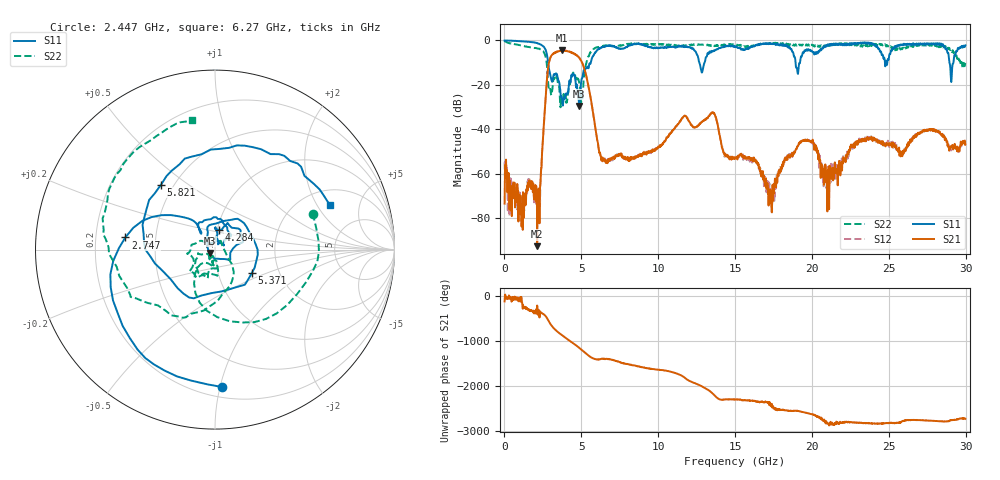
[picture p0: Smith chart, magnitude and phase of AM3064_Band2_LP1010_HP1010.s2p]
# Hz S DB R 50.0
!freq dBS11 angS11 dBS21 angS21 dBS12 angS12 dBS22 angS22
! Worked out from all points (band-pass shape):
!   1600 points, 10 MHz to 29.98 GHz, reference 50 ohm
!   highest |S21| = -4.55 dB at 3.759 GHz (marker M1); lowest = -92.6 dB at 2.128 GHz (marker M2)
!   |S21| within 3 dB of the highest: 3.001 GHz to 4.829 GHz (1.828 GHz wide, 46.7 % of centre)
!   lowest |S11| = -29.5 dB at 4.865 GHz (marker M3), VSWR 1.07, Z = 47.3 - j1.78 ohm
!   |S11| at or under -10 dB: 2.838 GHz to 5.615 GHz (2.777 GHz wide, 65.7 % of centre); 12.68 GHz to 13.02 GHz (341.4 MHz wide, 2.66 % of centre); 18.93 GHz to 19.22 GHz (289.4 MHz wide, 1.52 % of centre)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
!   |S22| runs from -30.1 to -0.3 dB; largest |S21 - S12| = 0.015
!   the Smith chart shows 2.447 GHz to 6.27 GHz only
!   S11 on the Smith chart (normalised r, x): 2.447 GHz: 0.27, -1.01; 2.747 GHz: 0.33, +0.06; 4.284 GHz: 1.02, +0.23; 5.371 GHz: 1.45, -0.41; 5.821 GHz: 0.43, +0.40; 6.27 GHz: 2.74, +2.59
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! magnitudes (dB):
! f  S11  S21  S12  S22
! 10 MHz  -0.1  -73.5  -54.9  -0.3
! 1.097 GHz  -0.4  -73.7  -81.3  -2.4
! 2.128 GHz  -1.2  -92.6  -78.1  -3.7
! 2.447 GHz  -2.3  -50.5  -50.9  -4.7
! 2.747 GHz  -5.9  -19.1  -19.1  -10.2
! 3.759 GHz  -27.0  -4.5  -4.6  -28.2
! 4.284 GHz  -19.0  -5.3  -5.1  -19.1
! 4.865 GHz  -29.5  -7.8  -7.8  -19.3
! 5.015 GHz  -17.5  -9.6  -9.5  -25.5
! 5.371 GHz  -12.3  -17.5  -17.5  -8.9
! 5.821 GHz  -6.5  -35.1  -35.1  -3.7
! 6.27 GHz  -3.3  -52.3  -52.5  -2.7
! 10 GHz  -3.4  -47.9  -47.7  -1.8
! 13.54 GHz  -5.1  -32.5  -32.4  -2.6
! 15 GHz  -2.6  -53.2  -53.3  -1.8
! 17.33 GHz  -1.3  -70.3  -69.4  -1.4
! 19.99 GHz  -4.7  -45.7  -46.0  -1.9
! 20.98 GHz  -2.2  -59.2  -58.0  -2.8
! 25 GHz  -8.3  -46.3  -46.1  -2.3
! 28.28 GHz  -1.3  -41.3  -41.3  -3.1
! 29.08 GHz  -17.5  -48.0  -49.3  -5.1
! 29.98 GHz  -2.3  -46.8  -45.3  -10.2
